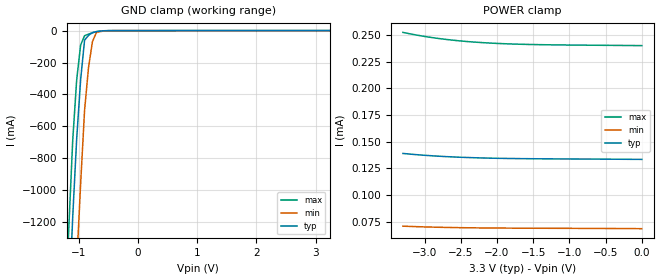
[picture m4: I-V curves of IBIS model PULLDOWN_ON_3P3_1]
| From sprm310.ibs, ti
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|BUFFER OPERATING IN NORMAL MODE
|   Model Cell PULLDOWN_ON_3P3
|PULLDOWN_ON_3P3
[Model]   PULLDOWN_ON_3P3_1
Model_type   Input
Polarity   Non-Inverting
Vinl =  0.8v
Vinh =  2v
C_comp   2.1697p   1.9812p   2.6822p
[Model Spec]
Vinl   0.8v   0.8v   0.8v
Vinh   2v   2v   2v
[Temperature Range]   25   125   -40
[Voltage Range]   3.3   3   3.6
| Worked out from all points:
|   GND clamp passes 1 mA (typ) near -0.56 V on its own axis
[POWER_clamp]
|   voltage   I(typ)   I(min)   I(max)
-3.3V     139.1uA    71.02uA    252.4uA
-3.2V     138.4uA    70.76uA    251uA
-3V       137.3uA    70.32uA    248.6uA
-2.9V     136.9uA    70.14uA    247.5uA
-2.7V     136.1uA    69.83uA    245.7uA
-2.6V     135.8uA    69.7uA     245uA
-2.4V     135.2uA    69.5uA     243.7uA
-2.1V     134.7uA    69.29uA    242.4uA
-1.8V     134.3uA    69.16uA    241.5uA
-1.4V     134.1uA    69.05uA    240.9uA
-1V       133.9uA    68.96uA    240.5uA
-11.55fV  133.5uA    68.67uA    240uA
[GND_clamp]
|   voltage   I(typ)   I(min)   I(max)
-3.3V     -22.4A     -23.17A    -21.98A
-1.233V   -2.327A    -3.192A    -1.823A
-1.167V   -1.741A    -2.598A    -1.245A
-1.1V     -1.17A     -2.014A    -689.7mA
-1.033V   -680.3mA   -1.468A    -310.2mA
-966.7mV  -310.2mA   -963.5mA   -90.96mA
-900mV    -59.69mA   -500.1mA   -31.9mA
-833.3mV  -29.95mA   -231.2mA   -22.02mA
-766.7mV  -12.14mA   -68.63mA   -13.53mA
-700mV    -6.252mA   -12.29mA   -6.425mA
-433.3mV  -117.8uA   -258.1uA   -108.7uA
3.233V    133.5uA    68.76uA    239.7uA
